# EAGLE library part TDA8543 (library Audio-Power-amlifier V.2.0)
2 W BTL audio amplifier
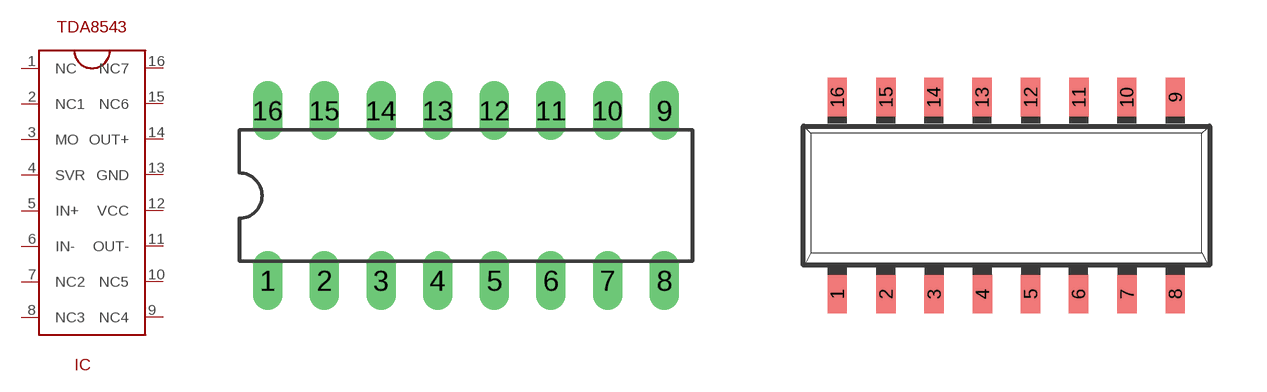
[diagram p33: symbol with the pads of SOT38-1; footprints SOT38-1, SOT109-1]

Designator prefix IC

## TDA8543  [SOT38-1]
1  NC  nc
2  NC1  nc
3  MO
4  SVR
5  IN+  in
6  IN-  in
7  NC2  nc
8  NC3  nc
9  NC4  nc
10  NC5  nc
11  OUT-  out
12  VCC  pwr
13  GND  pwr
14  OUT+  out
15  NC6  nc
16  NC7  nc

## TDA8543SOT109-1  [SOT109-1]
Pads as for SOT38-1

## Footprint SOT38-1 (pad centres in mm)
Dual In Line Package
drill 0.813 long: 1 -8.89,-3.81; 2 -6.35,-3.81; 3 -3.81,-3.81; 4 -1.27,-3.81; 5 1.27,-3.81; 6 3.81,-3.81; 7 6.35,-3.81; 8 8.89,-3.81; 9 8.89,3.81; 10 6.35,3.81; 11 3.81,3.81; 12 1.27,3.81; 13 -1.27,3.81; 14 -3.81,3.81; 15 -6.35,3.81; 16 -8.89,3.81

## Footprint SOT109-1 (pad centres in mm)
smd 0.508 x 1.016: 1 -4.45,-2.59; 2 -3.17,-2.59; 3 -1.9,-2.59; 4 -0.63,-2.59; 5 0.64,-2.59; 6 1.9,-2.59; 7 3.18,-2.59; 8 4.45,-2.59; 9 4.45,2.59; 10 3.17,2.59; 11 1.91,2.59; 12 0.64,2.59; 13 -0.64,2.59; 14 -1.91,2.59; 15 -3.17,2.59; 16 -4.45,2.59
